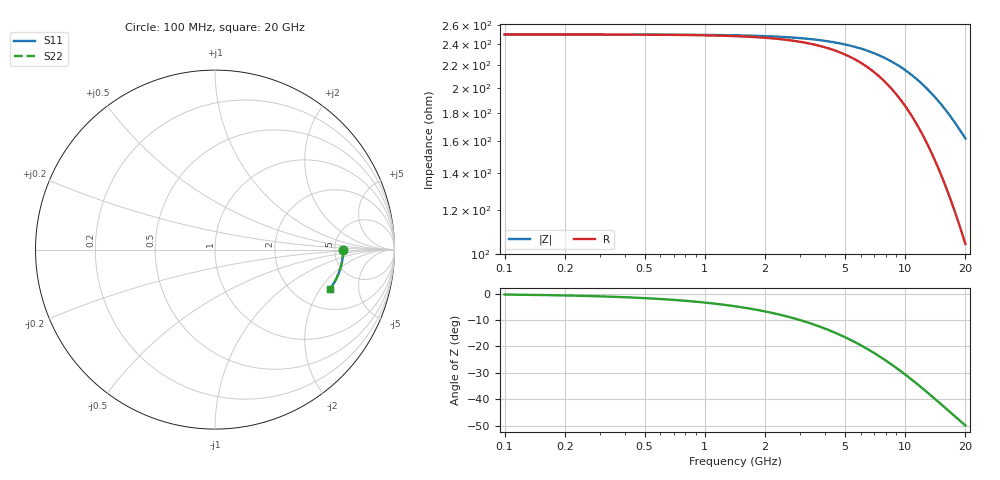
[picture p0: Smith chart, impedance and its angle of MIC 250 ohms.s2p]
! Vishay ElectroFilms Inc.
! MIC001 2500A - 250 Ohm in Series Configuration
! March 2012
# GHz S MA R 50
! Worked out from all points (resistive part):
!   233 points, 100 MHz to 20 GHz, reference 50 ohm
!   read as one part in series: R = 250 ohm at 102.3 MHz
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0.1  0.7143 -0.1  0.2857 0.2  0.2857 0.2  0.7143 -0.1
0.2436751  0.7143 -0.2  0.2857 0.6  0.2857 0.6  0.7143 -0.2
0.3936352  0.7143 -0.4  0.2858 1.0  0.2858 1.0  0.7143 -0.4
0.5937753  0.7143 -0.6  0.2859 1.4  0.2859 1.4  0.7143 -0.6
0.9375335  0.7142 -0.9  0.2861 2.3  0.2861 2.3  0.7142 -0.9
1.414214  0.7141 -1.4  0.2866 3.4  0.2866 3.4  0.7141 -1.4
1.818091  0.714 -1.8  0.2872 4.4  0.2872 4.4  0.714 -1.8
2.284535  0.7138 -2.2  0.2881 5.5  0.2881 5.5  0.7138 -2.2
2.805834  0.7135 -2.7  0.2893 6.7  0.2893 6.7  0.7135 -2.7
3.446086  0.7131 -3.3  0.291 8.2  0.291 8.2  0.7131 -3.3
4.430234  0.7124 -4.3  0.2945 10.4  0.2945 10.4  0.7124 -4.3
5.695439  0.7111 -5.5  0.3 13.1  0.3 13.1  0.7111 -5.5
6.995058  0.7095 -6.7  0.3069 15.7  0.3069 15.7  0.7095 -6.7
8.397251  0.7074 -8.1  0.3156 18.3  0.3156 18.3  0.7074 -8.1
9.413006  0.7057 -9.0  0.3227 20.1  0.3227 20.1  0.7057 -9.0
10.55163  0.7035 -10.1  0.3312 21.9  0.3312 21.9  0.7035 -10.1
11.82798  0.7008 -11.3  0.3415 23.7  0.3415 23.7  0.7008 -11.3
12.95936  0.6982 -12.3  0.3512 25.2  0.3512 25.2  0.6982 -12.3
14.19896  0.6952 -13.5  0.3623 26.6  0.3623 26.6  0.6952 -13.5
15.9165  0.6905 -15.1  0.3784 28.3  0.3784 28.3  0.6905 -15.1
17.84181  0.6847 -16.8  0.3971 29.9  0.3971 29.9  0.6847 -16.8
20  0.6777 -18.7  0.4187 31.2  0.4187 31.2  0.6777 -18.7
